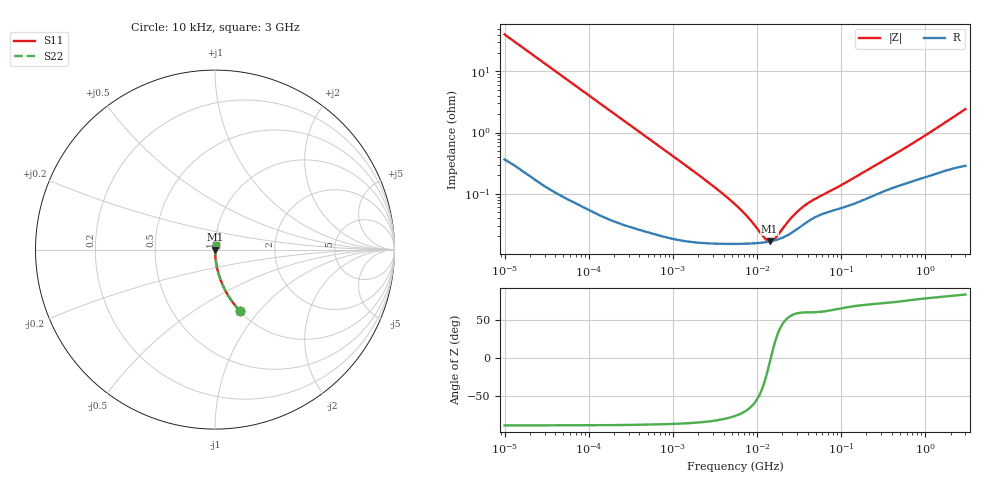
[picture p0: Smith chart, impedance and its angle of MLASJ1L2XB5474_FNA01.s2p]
! MLASJ1L2XB5474_FNA01  S-PARAMETER MODEL  ( Standard Model )
! Model Generated by TAIYO YUDEN Corporation (http://www.ty-top.com)
! Version 1.0
! TAIYO YUDEN Control No. 220601
! Copyright(c) 2010 TAIYO YUDEN CO.,LTD. All Rights Reserved.
! Product Description (link to TY-COMPAS)
! https://ds.yuden.co.jp/TYCOMPAS/or/detail?pn=MLASJ1L2XB5474KFNA01&u=M
! Products Name : Multilayer Ceramic Capacitors
! Characteristics :
!  Capacitance : 0.47 [uF] , Rated Voltage : 6.3 [V] , TCC : X5R
!  Case Size : 1.0 x 0.5 / 0.039 x 0.02 [mm/inch] , Thickness : 0.2 / 0.008 [mm/inch]
!  (Conditions: Temperature = 25 [degC] , DC Bias Voltage = 0 [V])
! External Node Assignments :
!  1  o---| |---o  2
! GND o---------o GND
! Frequency Range : 10kHz  -  3GHz  [ 401 STEP ]
# MHZ S RI R 50
! Freq[MHz].  S11 Real  S11 Imag  S21 Real  S21 Imag  S12 Real  S12 Imag  S22 Real  S22 Imag
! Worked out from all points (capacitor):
!   401 points, 10 kHz to 3 GHz, reference 50 ohm
!   read as one part in series: C = 395 nF near 10.65 kHz
!   lowest |Z| = 16.7 mohm at 14.1 MHz (marker M1)
!   series resonance near 14.62 MHz, so ESL is about 300 pH
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0.01  0.1417 -0.3443  0.8583 0.3443  0.8583 0.3443  0.1417 -0.3443
0.016047  0.0616 -0.2356  0.9384 0.2356  0.9384 0.2356  0.0616 -0.2356
0.027426  0.0227 -0.1442  0.9773 0.1442  0.9773 0.1442  0.0227 -0.1442
0.045421  0.00886 -0.0886  0.9911 0.0886  0.9911 0.0886  0.00886 -0.0886
0.082683  0.00304 -0.0491  0.997 0.0491  0.997 0.0491  0.00304 -0.0491
0.199902  0.000771 -0.0205  0.9992 0.0205  0.9992 0.0205  0.000771 -0.0205
0.683653  0.000244 -0.00604  0.9998 0.00604  0.9998 0.00604  0.000244 -0.00604
2.652321  0.000156 -0.00152  0.9998 0.00152  0.9998 0.00152  0.000156 -0.00152
5.477226  0.000152 -0.000656  0.9998 0.000656  0.9998 0.000656  0.000152 -0.000656
7.996027  0.000153 -0.000367  0.9998 0.000367  0.9998 0.000367  0.000153 -0.000367
12.43293  0.000161 -9.35e-05  0.9998 9.35e-05  0.9998 9.35e-05  0.000161 -9.35e-05
14.10408  0.000165 -2.05e-05  0.9998 2.05e-05  0.9998 2.05e-05  0.000165 -2.05e-05
15.02209  0.000168 1.58e-05  0.9998 -1.58e-05  0.9998 -1.58e-05  0.000168 1.58e-05
16.51234  0.000174 7.05e-05  0.9998 -7.05e-05  0.9998 -7.05e-05  0.000174 7.05e-05
24.10585  0.000217 0.000296  0.9998 -0.000296  0.9998 -0.000296  0.000217 0.000296
30.05882  0.000265 0.000432  0.9997 -0.000432  0.9997 -0.000432  0.000265 0.000432
36.31858  0.00032 0.000544  0.9997 -0.000544  0.9997 -0.000544  0.00032 0.000544
45.28751  0.000389 0.000668  0.9996 -0.000668  0.9996 -0.000668  0.000389 0.000668
106.0924  0.000598 0.00131  0.9994 -0.00131  0.9994 -0.00131  0.000598 0.00131
374.4521  0.0012 0.00376  0.9988 -0.00376  0.9988 -0.00376  0.0012 0.00376
798.0379  0.00173 0.00717  0.9983 -0.00717  0.9983 -0.00717  0.00173 0.00717
3000  0.00343 0.024  0.9966 -0.024  0.9966 -0.024  0.00343 0.024
